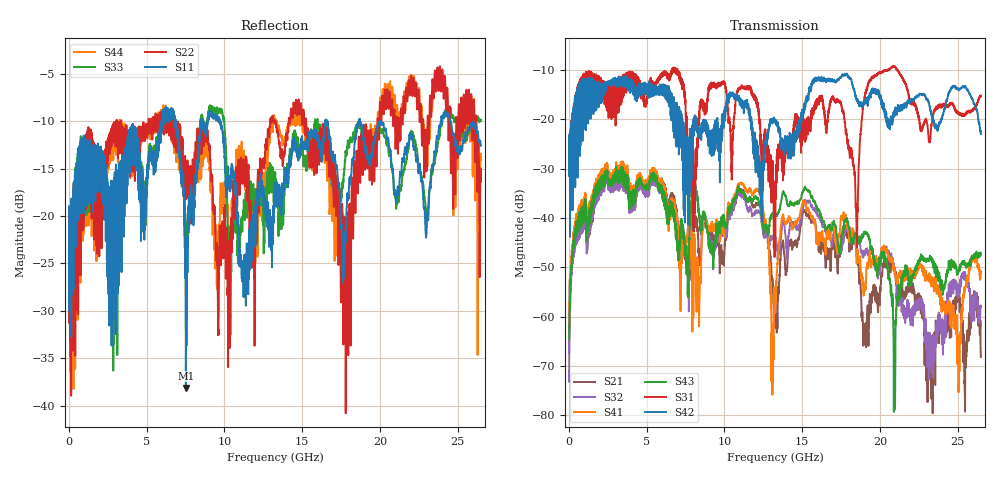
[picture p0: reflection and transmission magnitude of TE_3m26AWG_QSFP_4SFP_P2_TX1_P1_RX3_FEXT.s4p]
!Agilent Technologies,N5222A,MY51421691,A.10.00.00
!Agilent N5222A: A.10.00.00
!Date: Friday, January 30, 2015 12:36:53
!Correction: S11(Full 4 Port(1,2,3,4))
!S12(Full 4 Port(1,2,3,4))
!S13(Full 4 Port(1,2,3,4))
!S14(Full 4 Port(1,2,3,4))
!S21(Full 4 Port(1,2,3,4))
!S22(Full 4 Port(1,2,3,4))
!S23(Full 4 Port(1,2,3,4))
!S24(Full 4 Port(1,2,3,4))
!S31(Full 4 Port(1,2,3,4))
!S32(Full 4 Port(1,2,3,4))
!S33(Full 4 Port(1,2,3,4))
!S34(Full 4 Port(1,2,3,4))
!S41(Full 4 Port(1,2,3,4))
!S42(Full 4 Port(1,2,3,4))
!S43(Full 4 Port(1,2,3,4))
!S44(Full 4 Port(1,2,3,4))
!S4P File: Measurements: <S11,S12,S13,S14>,
!<S21,S22,S23,S24>,
!<S31,S32,S33,S34>,
!<S41,S42,S43,S44>:
# Hz S  dB  R 50.0
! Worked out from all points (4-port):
!   2650 points, 10 MHz to 26.5 GHz, reference 50 ohm
!   strongest paths, dB at 10 MHz, 6.63 GHz, 13.26 GHz, 19.88 GHz, 26.5 GHz:
!     S42: -25.0, -15.8, -20.0, -14.0, -23.0
!     S31: -24.9, -10.3, -36.3, -10.7, -15.2
!     S43: -64.6, -38.7, -38.9, -50.1, -47.4
!     S41: -63.3, -37.7, -55.8, -49.4, -51.2
!     S32: -73.2, -38.0, -43.6, -51.7, -58.0
!     S21: -67.4, -36.6, -57.4, -58.8, -68.1
!   lowest |S11| = -38.1 dB at 7.52 GHz (marker M1), VSWR 1.03, Z = 51.2 + j0.311 ohm
!   |S11| at or under -10 dB: start of sweep to 5.956 GHz; 9.719 GHz to 16.5 GHz (6.777 GHz wide, 51.7 % of centre); 20.05 GHz to 23.92 GHz (3.865 GHz wide, 17.6 % of centre)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
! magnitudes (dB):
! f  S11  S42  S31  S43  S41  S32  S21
! 10 MHz  -19.0  -25.0  -24.9  -64.6  -63.3  -73.2  -67.4
! 2.38 GHz  -16.3  -12.5  -13.1  -32.2  -31.0  -33.0  -32.1
! 7.52 GHz  -38.1  -23.6  -19.8  -46.8  -44.0  -45.3  -47.6
! 17.33 GHz  -16.7  -11.9  -16.4  -46.0  -43.7  -45.4  -47.8
! 18.49 GHz  -11.1  -15.7  -41.9  -43.7  -47.3  -43.2  -47.2
! 19.59 GHz  -12.2  -14.4  -11.4  -48.0  -48.2  -47.5  -53.7
! 26.5 GHz  -12.6  -23.0  -15.2  -47.4  -51.2  -58.0  -68.1
